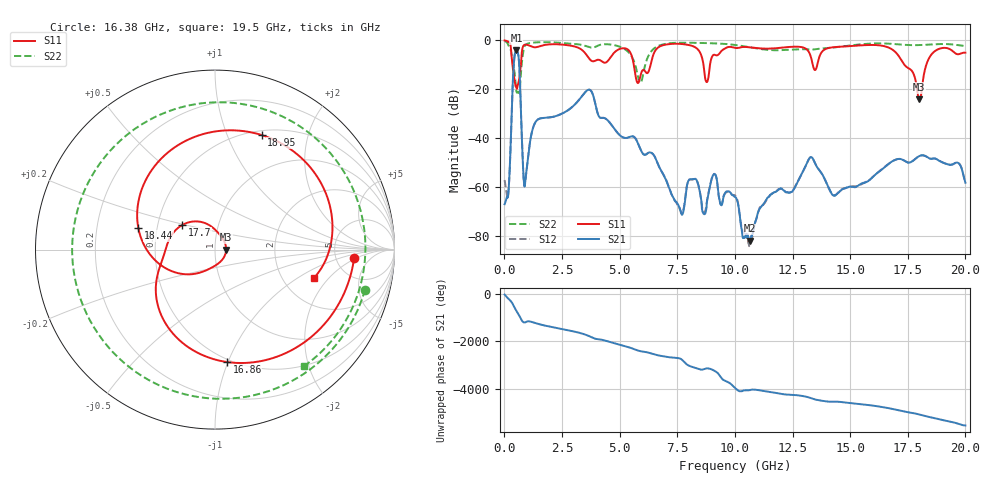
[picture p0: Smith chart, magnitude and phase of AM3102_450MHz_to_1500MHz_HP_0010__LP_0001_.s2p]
!Agilent Technologies,E8364B,MY43040894,A.07.50.67
!Agilent E8364B: A.07.50.67
!Date: Thursday, January 11, 2018 05:23:53
!Correction: S11(Full 2 Port(1,2))
!S21(Full 2 Port(1,2))
!S12(Full 2 Port(1,2))
!S22(Full 2 Port(1,2))
!S2P File: Measurements: S11, S21, S12, S22:
# Hz S  dB  R 50
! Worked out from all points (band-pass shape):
!   1601 points, 10 MHz to 20 GHz, reference 50 ohm
!   highest |S21| = -4.17 dB at 522.2 MHz (marker M1); lowest = -82.0 dB at 10.64 GHz (marker M2)
!   |S21| within 3 dB of the highest: 433 MHz to 620 MHz (187 MHz wide, 35.5 % of centre)
!   lowest |S11| = -24.2 dB at 18 GHz (marker M3), VSWR 1.13, Z = 56.6 + j0.0464 ohm
!   |S11| at or under -10 dB: 346.7 MHz to 715.5 MHz (368.8 MHz wide, 69.4 % of centre); 5.614 GHz to 6.343 GHz (729.9 MHz wide, 12.2 % of centre); 17.35 GHz to 18.3 GHz (950.8 MHz wide, 5.33 % of centre)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
!   |S22| runs from -21.5 to -0.3 dB; largest |S21 - S12| = 0.0022
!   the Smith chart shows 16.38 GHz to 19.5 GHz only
!   S11 on the Smith chart (normalised r, x): 16.38 GHz: 7.48, -1.84; 16.86 GHz: 0.48, -0.99; 17.7 GHz: 0.67, +0.19; 18.44 GHz: 0.39, +0.12; 18.95 GHz: 0.55, +1.34; 19.5 GHz: 2.99, -1.39
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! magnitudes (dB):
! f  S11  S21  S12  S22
! 10 MHz  -0.1  -67.1  -57.2  -0.3
! 184.9 MHz  -0.6  -61.2  -60.9  -2.3
! 522.2 MHz  -19.0  -4.2  -4.2  -20.9
! 897.1 MHz  -1.8  -58.7  -58.6  -2.1
! 1.384 GHz  -2.8  -33.0  -33.0  -0.8
! 3.346 GHz  -3.8  -23.1  -23.1  -1.9
! 5.895 GHz  -14.9  -44.4  -44.4  -17.5
! 6.682 GHz  -2.9  -51.2  -51.1  -2.3
! 7.681 GHz  -1.5  -71.1  -70.8  -1.0
! 10.01 GHz  -3.1  -64.1  -63.5  -1.9
! 10.64 GHz  -2.9  -82.0  -83.9  -2.8
! 13.34 GHz  -8.4  -48.0  -48.0  -3.8
! 14.3 GHz  -2.8  -63.6  -63.6  -2.9
! 16.38 GHz  -2.2  -52.9  -52.8  -1.3
! 16.68 GHz  -3.0  -50.6  -50.5  -1.4
! 16.86 GHz  -4.0  -49.3  -49.4  -1.5
! 17.7 GHz  -12.8  -49.5  -49.5  -2.0
! 18 GHz  -24.2  -47.4  -47.4  -2.0
! 18.44 GHz  -7.1  -48.4  -48.4  -1.8
! 18.95 GHz  -3.2  -49.8  -49.7  -1.5
! 19.5 GHz  -4.8  -50.5  -50.6  -1.8
! 20 GHz  -5.1  -58.3  -58.5  -2.3
